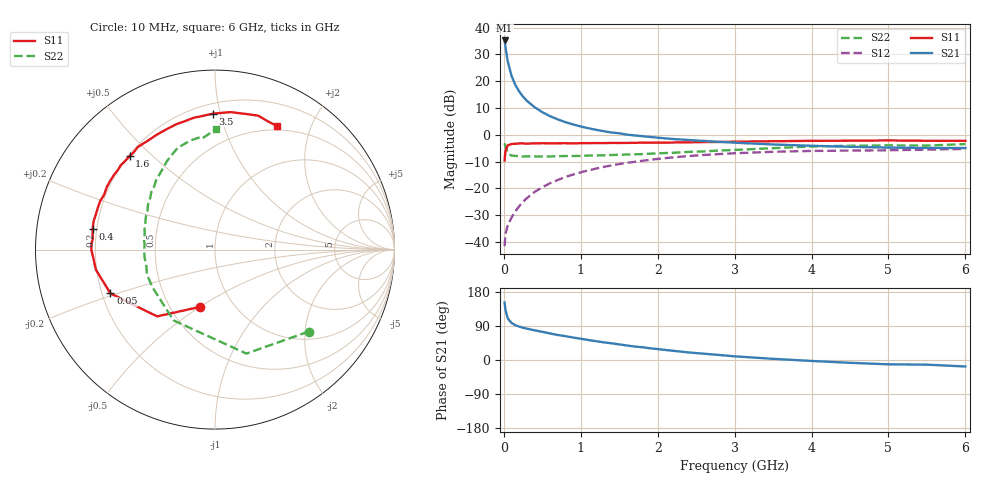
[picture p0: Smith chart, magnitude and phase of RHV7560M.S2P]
! SIEMENS Small Signal Semiconductors
! BFR106
! Si NPN RF Bipolar Junction Transistor in SOT23
! VCE = 0.75 V  IC = 60 mA
! Common Emitter S-Parameters:  August  1996
# GHz  S  MA  R  50
!  f  S11  S21  S12  S22
! GHz  MAG  ANG  MAG  ANG  MAG  ANG  MAG  ANG
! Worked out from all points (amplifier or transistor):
!   36 points, 10 MHz to 6 GHz, reference 50 ohm
!   highest |S21| = 35.2 dB at 10 MHz (marker M1)
!   |S21| within 3 dB of that: start of sweep to 24.3 MHz
!   unconditionally stable (mu >= 1): 127.5 MHz to end of sweep
!   at 250 MHz: K = 1.14, MAG = 17.4 dB, |S12| = -25.0 dB
!   at 1.4 GHz: K = 1.13, MAG = 3.9 dB, |S12| = -11.5 dB
!   at 6 GHz: K = 1.03, MAG = -1.0 dB, |S12| = -5.3 dB
!   S11 on the Smith chart (normalised r, x): 10 MHz: 0.70, -0.50; 50 MHz: 0.23, -0.19; 400 MHz: 0.18, +0.08; 1.6 GHz: 0.21, +0.42; 3.5 GHz: 0.27, +0.95; 6 GHz: 0.45, +1.53
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0.01  0.3302 -104.8  57.81 151.5  0.0083 67.0  0.6933 -41.2
0.02  0.4924 -130.9  44.86 133.3  0.0136 55.7  0.6052 -73.2
0.05  0.6318 -157.3  23.64 110.1  0.0203 50.5  0.4571 -120.4
0.1  0.6734 -170.5  12.59 97.6  0.0284 57.0  0.4069 -148.9
0.15  0.6802 -176.5  8.494 91.9  0.037 62.0  0.4038 -160.0
0.2  0.6885 -179.7  6.44 88.1  0.0465 65.3  0.3933 -166.4
0.25  0.689 177.1  5.138 85.1  0.056 66.9  0.3936 -171.0
0.3  0.6835 175.1  4.299 82.7  0.0656 68.5  0.3948 -173.8
0.4  0.6912 170.6  3.274 78.4  0.0854 69.3  0.3945 -178.5
0.5  0.6946 167.0  2.644 74.3  0.1047 69.0  0.3935 177.9
0.6  0.692 163.3  2.225 70.1  0.1241 67.9  0.3938 175.3
0.7  0.6935 159.8  1.942 66.1  0.143 66.6  0.3983 172.9
0.9  0.6893 153.6  1.559 59.3  0.1811 63.2  0.4009 167.7
1.1  0.6982 147.0  1.325 52.7  0.2163 59.7  0.4086 163.9
1.3  0.6994 140.8  1.166 46.5  0.2511 55.7  0.4143 159.5
1.6  0.7048 132.5  1.007 38.3  0.2985 50.0  0.4282 153.7
2.2  0.7173 117.1  0.833 24.3  0.3784 38.4  0.4608 141.7
3  0.7436 99.4  0.711 9.7  0.4517 24.1  0.5205 126.5
3.5  0.7575 90.8  0.659 3.1  0.4812 16.4  0.5626 118.2
4.5  0.7748 77.4  0.597 -7.4  0.5066 3.0  0.6226 102.9
5.5  0.7725 67.3  0.568 -12.3  0.5289 -4.8  0.6277 95.8
6  0.7709 63.3  0.565 -17.1  0.5442 -10.9  0.671 89.5
